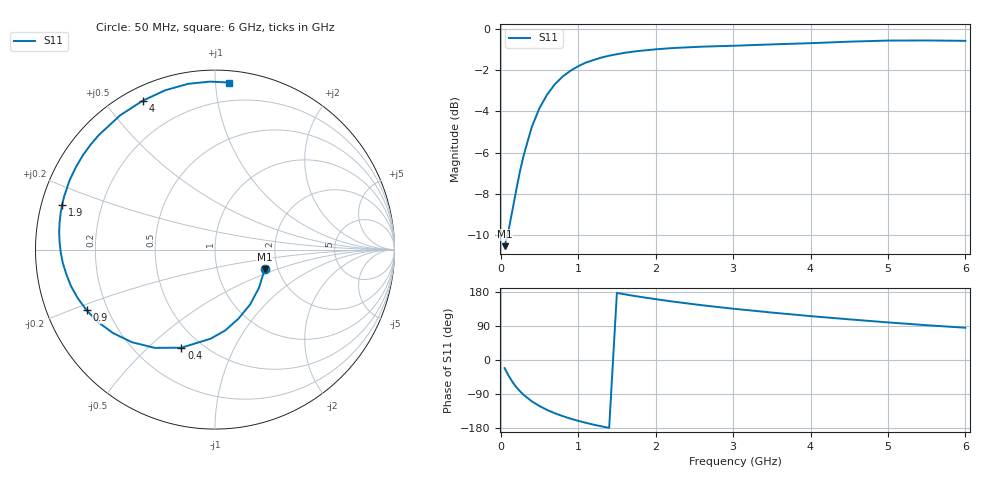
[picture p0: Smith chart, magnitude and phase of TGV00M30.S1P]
! SIEMENS Discrete & RF Semiconductors
! BAT64
! Si Schottky Diode in SOT23
! IF = 0.3 mA
! S-Parameters:  February  1997
# GHz  S  MA  R  50
!  f  S11
! GHz  MAG  ANG
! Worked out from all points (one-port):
!   34 points, 50 MHz to 6 GHz, reference 50 ohm
!   lowest |S11| = -10.5 dB at 50 MHz (marker M1), VSWR 1.85, Z = 85.2 - j20.4 ohm
!   |S11| at or under -10 dB: start of sweep to 85.02 MHz
!   S11 on the Smith chart (normalised r, x): 50 MHz: 1.70, -0.41; 400 MHz: 0.39, -0.64; 900 MHz: 0.12, -0.22; 1.9 GHz: 0.06, +0.14; 4 GHz: 0.06, +0.63; 6 GHz: 0.07, +1.09
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0.05  0.2978 -21.5
0.1  0.3245 -40.9
0.15  0.363 -57.4
0.2  0.4069 -71.4
0.25  0.4536 -82.7
0.3  0.497 -92.8
0.4  0.5776 -108.9
0.5  0.6422 -121.5
0.6  0.6932 -131.9
0.7  0.7341 -140.7
0.8  0.766 -148.1
0.9  0.7909 -154.7
1  0.8112 -160.5
1.1  0.8278 -165.8
1.2  0.84 -170.7
1.4  0.8601 -179.2
1.6  0.874 173.4
1.9  0.8873 163.6
2.2  0.8971 154.8
2.4  0.9009 149.6
2.6  0.9045 144.5
3  0.9091 135.4
3.5  0.916 125.2
4  0.9222 115.8
4.5  0.9301 107.3
5  0.9357 99.2
5.5  0.9363 91.8
6  0.9344 85.1
